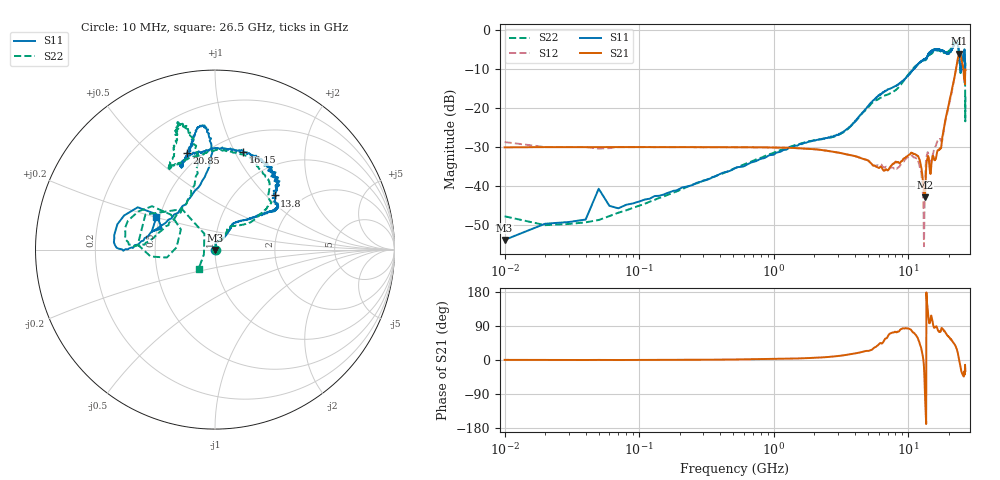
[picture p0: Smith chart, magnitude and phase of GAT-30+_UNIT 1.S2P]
!Created: 09-26-2013 at 09:17:33
!Mini-Circuits
!S2P DATA File Format
!Type: FIXED ATTENUATOR
!MODEL: GAT-30+
!S/N: Unit 1
!PIN OUT: PORT 1 - PIN 1, PORT 2 - PIN 3, GROUND - PIN 2,4
!TEST CONDITIONS: Z:50 OHM SYSTEM, INPUT POWER = -10dBm
!AP#: 130905
!PROD RUN: QM1142005 DATE CODE: 1142 WAFER/LOT#: WH461P005,AP130905
!REMARK: UNITS MOUNTED ON TB-154 D/C 1225. PORT EXTENSION HAS BEEN DONE.
!TESTED ON: NETWORK ANALYZER MODEL AG N5242A S/N 71932 CAL DUE DATE 3/15/14
! Frequency  S11 dB  S11 DEG  S21 dB  S21 DEG  S12 dB  S12 DEG  S22 dB  S22 DEG
# MHZ S DB R 50
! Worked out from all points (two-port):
!   930 points, 10 MHz to 26.5 GHz, reference 50 ohm
!   highest |S21| = -5.99 dB at 23.95 GHz (marker M1); lowest = -43.0 dB at 13.2 GHz (marker M2)
!   |S21| within 3 dB of the highest: 22.82 GHz to 25.32 GHz (2.498 GHz wide, 10.4 % of centre)
!   lowest |S11| = -53.9 dB at 10 MHz (marker M3), VSWR 1.00, Z = 50.1 - j0.182 ohm
!   |S11| at or under -10 dB: start of sweep to 10.92 GHz; 24.33 GHz to 24.79 GHz (453.8 MHz wide, 1.85 % of centre)
!   |S22| runs from -50.2 to -2.6 dB; largest |S21 - S12| = 0.026
!   S11 on the Smith chart (normalised r, x): 10 MHz: 1.00, -0.00; 13.8 GHz: 1.49, +1.12; 16.15 GHz: 0.68, +1.08; 20.85 GHz: 0.42, +0.66; 26.5 GHz: 0.48, +0.20
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10  -53.95 -64.8  -30.13 0.4  -28.77 5.8  -47.88 -39.9
40  -48.71 28.3  -30.09 0.0  -30.03 0.2  -49.43 19.1
140  -42.61 49.9  -30.07 0.2  -30.05 0.0  -43.18 55.6
520  -35.45 70.5  -30.11 1.4  -30.08 1.3  -35.41 73.4
1920  -28.49 84.6  -30.58 5.5  -30.60 5.6  -28.44 88.9
3260  -26.20 68.0  -31.72 12.1  -31.74 12.4  -26.35 71.0
7150  -15.12 55.2  -35.74 66.8  -35.74 57.9  -16.40 57.6
11500  -9.18 36.3  -32.07 62.7  -32.97 71.5  -9.02 38.3
12450  -7.94 32.9  -35.18 30.2  -36.62 49.8  -8.03 39.7
13000  -7.50 34.8  -41.31 -10.6  -50.94 -15.1  -7.75 40.0
13200  -7.37 34.2  -42.95 -65.0  -43.87 -160.8  -7.75 41.5
13450  -7.33 36.6  -37.87 -141.5  -34.48 166.0  -7.63 44.3
13800  -6.96 42.3  -33.25 146.1  -31.74 126.7  -6.97 47.8
14650  -5.71 51.6  -36.59 112.0  -34.88 105.9  -6.09 54.9
16150  -4.95 73.8  -32.28 89.1  -29.22 85.2  -5.20 77.3
17850  -5.26 101.9  -27.55 82.6  -28.28 67.6  -5.52 106.4
20850  -5.05 106.2  -15.92 53.2  -16.41 53.4  -4.40 112.5
22900  -3.17 94.8  -8.66 27.8  -8.71 28.2  -2.98 104.3
23950  -7.41 96.7  -5.99 -5.6  -6.10 -6.4  -7.48 104.6
24600  -10.45 139.4  -6.87 -26.8  -7.27 -27.5  -10.56 149.6
25750  -5.83 -179.3  -10.79 -43.6  -11.14 -40.4  -5.92 171.0
26500  -8.56 151.2  -10.22 -29.2  -10.49 -24.8  -17.03 -130.4
